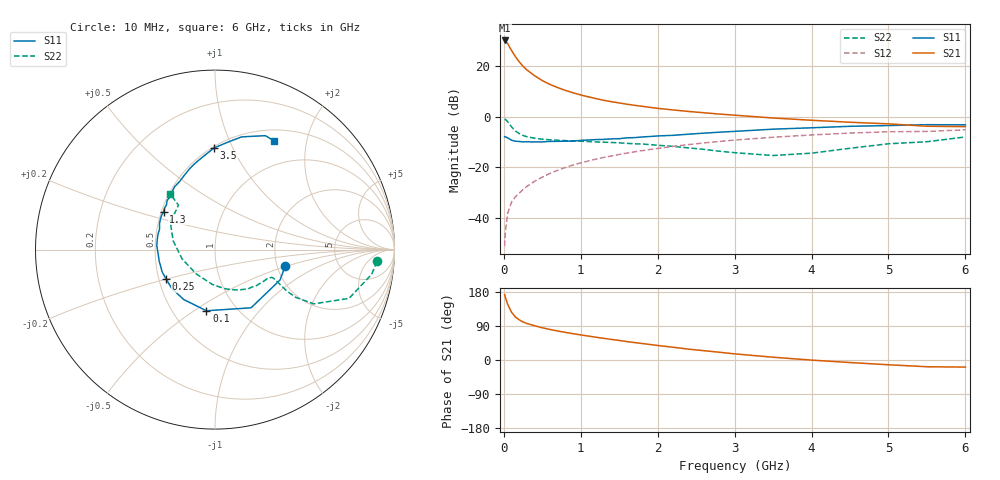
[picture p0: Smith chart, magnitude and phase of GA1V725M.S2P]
! Infineon Technologies  Discrete & RF Semiconductors
! BF775
! Si NPN RF Bipolar Junction Transistor in SOT23
! VCE = 1.75 V  IC = 25 mA
! Common Emitter S-Parameters:  May  1996
# GHz  S  MA  R  50
!  f  S11  S21  S12  S22
! GHz  MAG  ANG  MAG  ANG  MAG  ANG  MAG  ANG
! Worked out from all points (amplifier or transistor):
!   36 points, 10 MHz to 6 GHz, reference 50 ohm
!   highest |S21| = 30.0 dB at 10 MHz (marker M1)
!   |S21| within 3 dB of that: start of sweep to 82.33 MHz
!   unconditionally stable (mu >= 1): 207.1 MHz to end of sweep
!   at 250 MHz: K = 1.07, MAG = 22.6 dB, |S12| = -28.7 dB
!   at 1.4 GHz: K = 1.24, MAG = 7.7 dB, |S12| = -15.5 dB
!   at 6 GHz: K = 1.05, MAG = -0.8 dB, |S12| = -5.2 dB
!   S11 on the Smith chart (normalised r, x): 10 MHz: 2.21, -0.49; 100 MHz: 0.73, -0.56; 250 MHz: 0.55, -0.20; 1.3 GHz: 0.51, +0.25; 3.5 GHz: 0.51, +0.85; 6 GHz: 0.65, +1.49
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0.01  0.4019 -13.3  31.73 172.5  0.0028 85.6  0.9052 -4.2
0.02  0.3999 -25.1  31.1 165.2  0.0054 74.2  0.8834 -9.0
0.05  0.3815 -58.2  27.4 146.8  0.0125 72.1  0.7946 -20.0
0.1  0.344 -98.0  20.15 126.1  0.0207 64.2  0.6277 -28.8
0.15  0.3283 -122.1  15.21 113.6  0.0264 64.2  0.5223 -30.6
0.2  0.3237 -137.8  12.05 106.0  0.031 65.2  0.4635 -30.0
0.25  0.3183 -149.0  9.808 100.4  0.0367 66.3  0.4251 -28.8
0.3  0.3194 -157.1  8.324 96.3  0.0422 68.5  0.4021 -27.8
0.4  0.3174 -168.2  6.407 90.4  0.0533 69.8  0.375 -26.5
0.5  0.3184 -177.0  5.138 85.0  0.0641 70.6  0.3591 -26.0
0.6  0.3251 176.1  4.309 80.6  0.0761 70.9  0.3498 -26.3
0.7  0.3264 170.5  3.739 76.5  0.0877 70.6  0.3429 -27.3
0.8  0.3287 165.2  3.292 72.9  0.0993 69.6  0.3366 -28.4
1.1  0.3462 152.0  2.451 63.1  0.1341 67.6  0.3228 -33.2
1.3  0.3563 143.6  2.098 57.1  0.1573 65.6  0.3134 -37.0
1.7  0.386 130.6  1.673 46.0  0.2025 61.0  0.2918 -46.0
2.2  0.4282 117.3  1.354 33.7  0.2593 54.6  0.2594 -60.3
2.8  0.4934 103.0  1.124 20.5  0.3245 46.3  0.2084 -83.9
3.5  0.5663 90.6  0.94 7.3  0.3925 35.9  0.1712 -128.1
4.5  0.6449 76.8  0.775 -6.7  0.4745 21.2  0.238 168.2
5.5  0.6942 66.1  0.647 -17.8  0.5112 6.2  0.3203 129.4
6  0.6893 61.3  0.635 -18.7  0.55 2.0  0.3977 128.8
